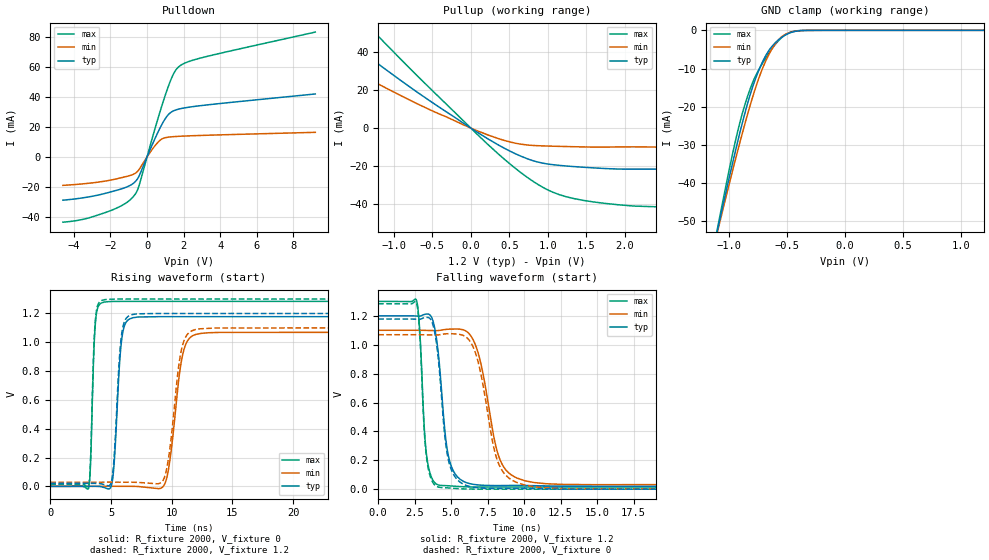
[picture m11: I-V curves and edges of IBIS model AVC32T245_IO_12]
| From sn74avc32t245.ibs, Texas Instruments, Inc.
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[Model]   AVC32T245_IO_12
Model_type  I/O
Vinl=0.385
Vinh=0.845
Enable   Active-Low
Vref =   0
Rref =   2000
Cref =   15p
Vmeas =   0.6
| variable   typ   min   max
C_comp   5.29pF   4.66pF   5.83pF
| C_pullup   5.78pF   3.89pF   7.84pF
| C_pulldown   5.32pF   4.76pF   7.02pF
| C_tri-state   5.29pF   4.66pF   5.83pF
[Temperature Range]   40   100   -40
| Ambient temperature   25   85   -40
[Voltage range]   1.2   1.1   1.3
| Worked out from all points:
|   slope of the pulldown table from 0 to 0.18 V, typ, clamps not added: 34.6 ohm
|   slope of the pullup table from 0 to 0.18 V, typ, clamps not added: 38.6 ohm
|   GND clamp passes 1 mA (typ) near -0.50 V on its own axis
|   rising waveform, R_fixture 2000, V_fixture 0: 20-80 % time 467ps typ, 865ps min, 282ps max; typ from 0 V to 1.18 V
|   falling waveform, R_fixture 2000, V_fixture 1.2: 20-80 % time 670ps typ, 1.21ns min, 399ps max; typ from 1.2 V to 0.02 V
|   rising waveform, R_fixture 2000, V_fixture 1.2: 20-80 % time 462ps typ, 847ps min, 279ps max; typ from 0.02 V to 1.2 V
|   falling waveform, R_fixture 2000, V_fixture 0: 20-80 % time 668ps typ, 1.21ns min, 398ps max; typ from 1.18 V to 0 V
[GND Clamp]
| AVC32T245_IO_12
|   Voltage   I(typ)   I(min)   I(max)
-4.6V     -597.8mA   -546.6mA   -662.5mA
-1.095V   -51.41mA   -51.9mA    -50.81mA
-1.07V    -47.97mA   -48.78mA   -46.93mA
-940mV    -30.76mA   -33.04mA   -28.1mA
-840mV    -18.99mA   -21.8mA    -17.13mA
-775mV    -12.84mA   -15.28mA   -12.1mA
-695mV    -7.204mA   -8.735mA   -7.744mA
-615mV    -3.665mA   -4.111mA   -4.191mA
-545mV    -1.809mA   -1.649mA   -1.862mA
-465mV    -549.4uA   -452.3uA   -430.6uA
-360mV    -50.53uA   -51.18uA   -21.62uA
1.2V      708.7pA    34.3nA     62.33pA
[Pulldown]
| AVC32T245_IO_12
|   Voltage   I(typ)   I(min)   I(max)
-4.6V     -28.79mA   -18.92mA   -43.46mA
-3.415V   -27.06mA   -17.81mA   -41.32mA
-2.03V    -23.44mA   -15.52mA   -35.94mA
-1.165V   -20.28mA   -13.12mA   -30.82mA
-680mV    -16.87mA   -11.13mA   -25.38mA
-435mV    -12.68mA   -8.327mA   -19.06mA
440mV     12.38mA    7.543mA    19.04mA
955mV     24.67mA    12.69mA    39.57mA
1.42V     30.53mA    13.49mA    54.64mA
1.79V     32.04mA    13.78mA    60.61mA
3.17V     34.51mA    14.41mA    66.63mA
9.2V      41.96mA    16.4mA     83.17mA
[Pullup]
| AVC32T245_IO_12
|   Voltage   I(typ)   I(min)   I(max)
-4.6V     40.24mA    7.956mA    186.3mA
-4.08V    45.4mA     8.808mA    167.8mA
-3.73V    53.62mA    9.647mA    154.2mA
-2.685V   79.31mA    16.98mA    111.4mA
-2.57V    75.87mA    21.96mA    106.5mA
-2.565V   75.72mA    49.42mA    106.3mA
-1.845V   53.66mA    37.03mA    75.82mA
-1.36V    38.76mA    26.71mA    55.3mA
575mV     -13.51mA   -7.977mA   -21.19mA
1.01V     -19.08mA   -9.527mA   -32.92mA
1.455V    -20.71mA   -9.971mA   -38.21mA
9.2V      -28.28mA   -12.48mA   -52.65mA
[Ramp]
| AVC32T245_IO_12
| variable   typ   min   max
dV/dt_r   0.72/4.81E-10   0.65/8.80E-10   0.78/2.90E-10
dV/dt_f   0.72/6.78E-10   0.65/1.22E-09   0.78/4.10E-10
R_load = 2000
[Rising Waveform]
| AVC32T245_IO_12
R_fixture =   2000
C_fixture =   0
L_fixture =   0
V_fixture =   0
V_fixture_min = 0
V_fixture_max = 0
|   Time   V(typ)   V(min)   V(max)
0s        18.11nV    102nV      416.8pV
3.155ns   608.7uV    -112.2uV   -13.83mV
3.69ns    448.5uV    152.3uV    1.106V
4.21ns    -2.723mV   127.2uV    1.273V
5.105ns   34.06mV    467.8uV    1.283V
5.83ns    982.1mV    362.3uV    1.284V
6.525ns   1.162V     267.3uV    1.284V
9.455ns   1.178V     21.9mV     1.284V
11.73ns   1.178V     1.046V     1.284V
29.99ns   1.178V     1.069V     1.284V
[Falling Waveform]
| AVC32T245_IO_12
R_fixture =   2000
C_fixture =   0
L_fixture =   0
V_fixture =   1.2
V_fixture_min = 1.1
V_fixture_max = 1.3
|   Time   V(typ)   V(min)   V(max)
0s        1.2V       1.1V       1.3V
2.635ns   1.198V     1.1V       1.304V
3.3ns     1.212V     1.099V     249.5mV
4.075ns   980.8mV    1.098V     31.14mV
4.815ns   228.7mV    1.107V     23.54mV
6.03ns    45.79mV    1.094V     16.13mV
6.94ns    28.68mV    910.8mV    14.76mV
8.265ns   25.01mV    226.6mV    14.53mV
9.515ns   25.97mV    76.79mV    14.51mV
29.99ns   20.14mV    28.8mV     14.5mV
[Rising Waveform]
| AVC32T245_IO_12
R_fixture =   2000
C_fixture =   0
L_fixture =   0
V_fixture =   1.2
V_fixture_min = 1.1
V_fixture_max = 1.3
|   Time   V(typ)   V(min)   V(max)
0s        20.14mV    28.74mV    14.5mV
3.155ns   20.71mV    28.68mV    2.227mV
3.685ns   20.46mV    28.94mV    1.125V
4.2ns     17.47mV    28.89mV    1.289V
5.08ns    51.99mV    29.12mV    1.299V
5.815ns   1.013V     28.88mV    1.3V
6.505ns   1.185V     28.69mV    1.3V
9.375ns   1.2V       55.91mV    1.3V
11.61ns   1.2V       1.078V     1.3V
29.99ns   1.2V       1.1V       1.3V
[Falling Waveform]
| AVC32T245_IO_12
R_fixture =   2000
C_fixture =   0
L_fixture =   0
V_fixture =   0
V_fixture_min = 0
V_fixture_max = 0
|   Time   V(typ)   V(min)   V(max)
0s        1.178V     1.069V     1.284V
2.635ns   1.177V     1.069V     1.287V
3.295ns   1.189V     1.068V     234.7mV
4.03ns    983.5mV    1.068V     17.73mV
4.79ns    212.5mV    1.076V     8.743mV
6.015ns   26.33mV    1.054V     1.403mV
6.86ns    9.258mV    877.4mV    252.2uV
8.16ns    4.995mV    201.5mV    30.57uV
9.445ns   5.821mV    48.62mV    10.14uV
29.99ns   161.1nV    39.78uV    -988.6pV
